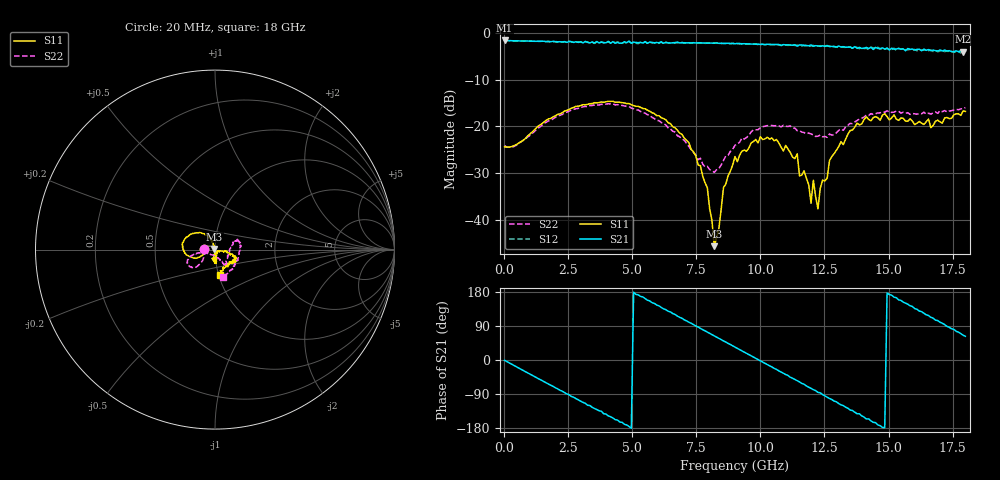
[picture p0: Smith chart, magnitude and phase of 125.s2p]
!Agilent Technologies,N5230A,US43500223,A.07.50.48
!Agilent N5230A: A.07.50.48
!Date: Monday, January 11, 2016 21:18:21
!Correction: S11(Full 2 Port(1,2))
!S21(Full 2 Port(1,2))
!S12(Full 2 Port(1,2))
!S22(Full 2 Port(1,2))
!S2P File: Measurements: S11, S21, S12, S22:
# Hz S  dB  R 50
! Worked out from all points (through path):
!   201 points, 20 MHz to 18 GHz, reference 50 ohm
!   highest |S21| = -1.60 dB at 20 MHz (marker M1); lowest = -4.0 dB at 17.91 GHz (marker M2)
!   group delay of S21, straight-line fit = 101 ps
!   lowest |S11| = -45.7 dB at 8.201 GHz (marker M3), VSWR 1.01, Z = 49.7 + j0.412 ohm
!   |S11| at or under -10 dB: start of sweep to end of sweep
!   |S22| runs from -29.9 to -15.2 dB; largest |S21 - S12| = 0.063
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2e7  -24.40 179.3  -1.60 -0.8  -1.60 -0.9  -24.14 179.3
1.5483e9  -19.11 -154.7  -1.76 -56.9  -1.78 -57.5  -19.44 -137.0
3.0766e9  -15.36 -173.4  -2.13 -111.9  -2.07 -112.2  -15.83 -141.5
4.8746e9  -15.12 156.8  -1.74 -175.4  -1.84 -176.5  -15.75 -159.7
6.0433e9  -17.72 132.6  -2.10 143.0  -2.22 142.1  -18.77 -168.3
7.6615e9  -28.43 105.6  -2.11 83.3  -2.21 82.0  -26.84 -143.3
7.9312e9  -33.17 98.8  -2.17 73.6  -2.18 72.2  -28.58 -130.2
8.2009e9  -45.68 127.2  -2.18 63.8  -2.18 62.1  -29.86 -105.0
8.5605e9  -33.14 -74.1  -2.22 50.4  -2.25 48.8  -27.32 -76.0
9.01e9  -26.48 -82.3  -2.32 34.0  -2.31 32.0  -24.05 -63.2
1.04484e10  -22.49 -88.9  -2.47 -18.2  -2.50 -20.8  -19.83 -58.4
1.14373e10  -25.88 -98.8  -2.83 -54.8  -2.63 -56.5  -20.94 -46.7
1.15272e10  -30.63 -100.2  -2.57 -57.8  -2.67 -60.4  -20.93 -42.4
1.19767e10  -36.48 -53.1  -2.56 -74.9  -2.79 -76.3  -21.63 -31.3
1.20666e10  -31.55 -61.2  -2.83 -78.2  -2.67 -80.4  -21.86 -27.8
1.22464e10  -37.68 -39.6  -2.77 -85.3  -2.80 -86.2  -22.12 -25.0
1.24262e10  -31.54 -24.4  -2.74 -91.2  -2.83 -93.4  -22.24 -16.8
1.31454e10  -23.28 -8.5  -3.01 -118.4  -2.98 -120.1  -20.59 8.1
1.50333e10  -18.62 -28.6  -3.64 172.6  -3.61 169.9  -16.96 16.3
1.66515e10  -20.28 -56.4  -3.78 112.7  -3.68 108.6  -17.38 -36.8
1.79101e10  -16.69 -77.5  -4.02 65.5  -4.00 62.4  -16.18 -71.5
1.8e10  -16.80 -79.9  -3.92 62.6  -4.23 58.9  -15.98 -73.6
